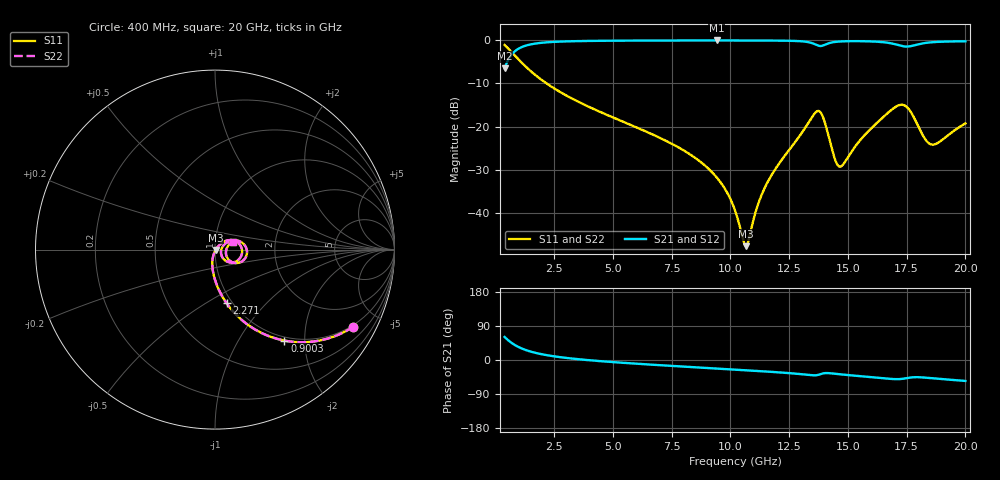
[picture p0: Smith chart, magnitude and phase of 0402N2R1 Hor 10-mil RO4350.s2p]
# GHz S MA R 50
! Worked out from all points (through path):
!   1960 points, 400 MHz to 20 GHz, reference 50 ohm
!   highest |S21| = -0.03 dB at 9.415 GHz (marker M1); lowest = -6.5 dB at 400 MHz (marker M2)
!   group delay of S21, straight-line fit = 11.3 ps
!   lowest |S11| = -47.7 dB at 10.67 GHz (marker M3), VSWR 1.01, Z = 50.4 - j0.205 ohm
!   |S11| at or under -10 dB: 2.189 GHz to end of sweep
!   |S22| runs from -47.7 to -1.1 dB; largest |S21 - S12| = 0
!   S11 on the Smith chart (normalised r, x): 400 MHz: 0.94, -3.61; 900.3 MHz: 0.94, -1.60; 2.271 GHz: 0.94, -0.62; 20 GHz: 1.21, +0.11
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0.4  0.8815 -29.2  0.4719 60.8  0.4719 60.8  0.8815 -29.2
0.9002552  0.6372 -52.7  0.77 37.3  0.77 37.3  0.6372 -52.7
1.460541  0.4517 -66.8  0.8911 23.1  0.8911 23.1  0.4517 -66.8
2.270955  0.3054 -77.8  0.9508 11.9  0.9508 11.9  0.3054 -77.8
3.671669  0.1862 -88.2  0.9806 1.3  0.9806 1.3  0.1862 -88.2
6.943338  0.07556 -101.6  0.9944 -13.5  0.9944 -13.5  0.07556 -101.6
8.424094  0.0451 -105.2  0.9957 -18.9  0.9957 -18.9  0.0451 -105.2
9.414599  0.02597 -105.2  0.996 -22.5  0.996 -22.5  0.02597 -105.2
10.205  0.01063 -94.8  0.9958 -25.4  0.9958 -25.4  0.01063 -94.8
10.66524  0.00413 -29.5  0.9954 -27.1  0.9954 -27.1  0.00413 -29.5
11.1855  0.01273 38.9  0.9947 -29.0  0.9947 -29.0  0.01273 38.9
11.5657  0.02221 45.1  0.9938 -30.5  0.9938 -30.5  0.02221 45.1
13.46667  0.1279 20.0  0.9299 -40.3  0.9299 -40.3  0.1279 20.0
13.69678  0.1511 -1.5  0.8765 -39.8  0.8765 -39.8  0.1511 -1.5
13.87688  0.1411 -24.6  0.861 -36.6  0.861 -36.6  0.1411 -24.6
14.45717  0.04158 -35.2  0.9578 -36.3  0.9578 -36.3  0.04158 -35.2
14.67728  0.03445 -7.7  0.9694 -37.8  0.9694 -37.8  0.03445 -7.7
16.73834  0.1472 17.8  0.9332 -49.4  0.9332 -49.4  0.1472 17.8
17.46871  0.1722 -18.4  0.8462 -48.2  0.8462 -48.2  0.1722 -18.4
18.28913  0.07166 -28.1  0.931 -46.5  0.931 -46.5  0.07166 -28.1
18.57928  0.06199 -9.9  0.9498 -48.0  0.9498 -48.0  0.06199 -9.9
20  0.109 24.5  0.9739 -55.2  0.9739 -55.2  0.109 24.5
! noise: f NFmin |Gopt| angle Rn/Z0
0.4  0.001262  0.7952  4.001  0.001272
2.571  0.005044  0.678  7.867  0.003013
4.752  0.008065  0.6377  13.04  0.004146
6.933  0.01091  0.6168  18.29  0.005172
9.104  0.01401  0.6128  23.44  0.006454
11.29  0.01931  0.6484  28.53  0.00982
13.47  0.0759  0.88  33.85  0.1254
15.64  0.04539  0.7826  38.93  0.03816
17.82  0.124  0.9048  44.11  0.2456
20  0.04926  0.7567  48.8  0.0341
